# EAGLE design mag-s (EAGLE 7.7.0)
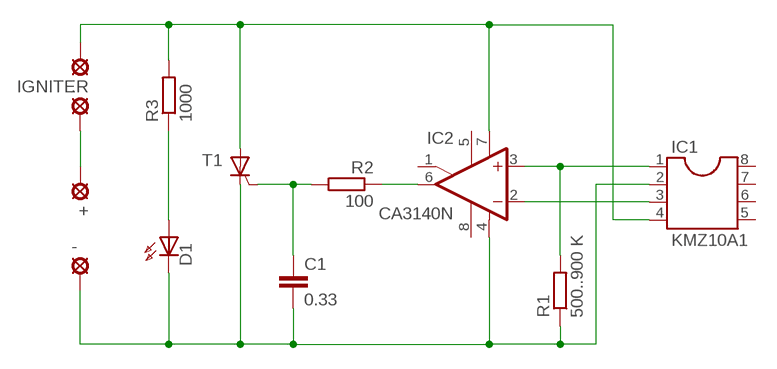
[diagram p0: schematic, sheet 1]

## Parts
+  SE11  [SE11]
-  SE11  [SE11]
.  SE11  [SE11]
C1  0.33  C-EUC0805K  [C0805K]
D1  HLMP6  [HLMP6]
IC1  KMZ10A1  DIL8  [DIL08]
IC2  CA3140N  [DIL08]
IGNITER  SE11  [SE11]
R1  500..900 K  R-EU_M0805  [M0805]
R2  100  R-EU_M0805  [M0805]
R3  1000  R-EU_M0805  [M0805]
T1  BT151  [TO220CL]

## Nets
N$2: IC1.4 IC2.7(V+) IGNITER.MP R3.2 T1.A
N$4: C1.1 R2.2 T1.G
N$5: D1.A R3.1
N$6: -.MP C1.2 D1.K IC1.2 IC2.4(V-) R1.1 T1.C
N$7: IC1.1 IC2.3(+IN) R1.2
N$8: +.MP ..MP
N$9: IC2.6(OUT) R2.1
N$10: IC1.3 IC2.2(-IN)
Unconnected: IC1.5 IC1.6 IC1.7 IC1.8 IC2.1(ON/CMP) IC2.5(ON) IC2.8(CMP)

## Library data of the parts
+ - . IGNITER = solpad:SE11: SOLDER PAD
C1 = rcl:C-EU: CAPACITOR, European symbol
D1 = display-hp:HLMP6: LED
IC1 = ic-package:DIL8: Dual In Line / Socket
IC2 = linear:CA3140: OP AMP
R1-R3 = rcl:R-EU_: RESISTOR, European symbol
T1 = triac:BT151: THYRISTOR

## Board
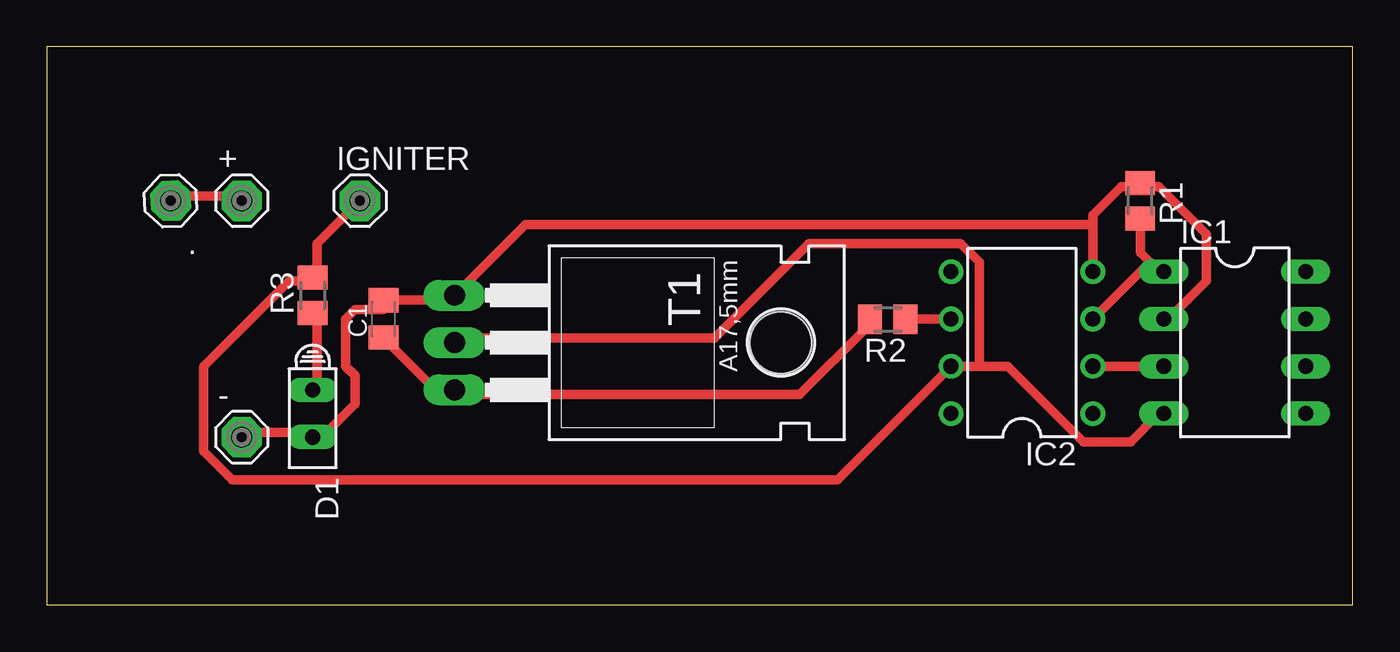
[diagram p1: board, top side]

Size 70.17 x 30.01 mm. Coordinates in mm from the lower left corner, seen from the top.
Outline: 0,0 70.17,0 70.17,30.01 0,30.01 0,0
Copper layers 1: Top 0.035mm
Design rules "default": minimum track width 20mil, minimum drill 20mil, track to track 20mil, track to pad 20mil, pad to pad 20mil, via to via 20mil, smd to smd 25mil, copper to edge 20mil, drill to drill 8mil, minimum pad ring 10mil, minimum via ring 8mil, stop-mask expansion 4mil, vias tented up to drill 0mil, thermal gap 10mil

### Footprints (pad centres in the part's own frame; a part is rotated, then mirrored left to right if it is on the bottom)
SE11 = drill 1.118 pad 2.159 octagon: MP 0,0
C0805K = smd 1.3 x 1.6: 1 -1,0; 2 1,0
HLMP6 = drill 0.813 long: A -1.27,0; K 1.27,0
DIL08 = drill 0.813 long: 1 -3.81,-3.81; 2 -1.27,-3.81; 3 1.27,-3.81; 4 3.81,-3.81; 5 3.81,3.81; 6 1.27,3.81; 7 -1.27,3.81; 8 -3.81,3.81
DIL08' = drill 0.813 pad 1.27: 1 -3.81,-3.81; 2 -1.27,-3.81; 3 1.27,-3.81; 4 3.81,-3.81; 5 3.81,3.81; 6 1.27,3.81; 7 -1.27,3.81; 8 -3.81,3.81
M0805 = smd 1.3 x 1.6: 1 -0.95,0; 2 0.95,0
TO220CL = drill 1.118 long: A 0,-6.35; C -2.54,-6.35; G 2.54,-6.35 | hole 3.302: 0,11.176

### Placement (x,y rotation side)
+  10.48,21.72 0 top
-  10.48,9.02 0 top
.  6.67,21.72 182.6 top
C1  18.1,15.37 90 top
D1  14.29,10.29 270 top
IC1  63.82,14.1 270 top
IC2  CA3140N  [DIL08']  52.39,14.1 90 top
IGNITER  16.83,21.72 0 top
R1  58.74,21.72 270 top
R2  45.18,15.35 180 top
R3  14.29,16.64 90 top
T1  28.26,14.1 270 top

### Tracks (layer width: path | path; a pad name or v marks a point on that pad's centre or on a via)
N$2
  Top 0.508: IGNITER.MP 14.54,19.43 14.54,17.91 R3.2 14.04,17.4 13.02,17.4 8.45,12.83 8.45,8.26 9.97,6.73 42.48,6.73 IC2.7 50.1,12.83 | 50.1,12.83 51.63,12.83 55.69,8.77 58.23,8.77 59.76,10.29 IC1.4 | 50.1,12.83 50.1,18.42 49.09,19.43 40.96,19.43 35.88,14.35 22.16,14.35 T1.A
N$4
  Top 0.508: C1.1 18.1,14.35 20.64,11.81 21.66,11.81 T1.G 22.16,11.31 40.45,11.31 44.01,14.86 R2.2
N$5
  Top 0.508: R3.1 14.54,15.37 14.54,11.81 D1.A
N$6
  Top 0.508: 58.74,22.48 57.72,22.48 56.2,20.96 56.2,20.45 | IC2.4 56.2,20.45 | 58.74,22.48 59.76,22.48 62.3,19.94 62.3,17.4 60.26,15.37 IC1.2 | 58.74,22.48 R1.1 | -.MP 10.48,9.27 14.04,9.27 D1.K 14.54,8.77 16.58,10.8 16.58,12.32 16.07,12.83 16.07,15.37 16.58,15.88 18.1,15.88 C1.2 18.1,16.39 21.66,16.39 T1.C 25.72,20.45 56.2,20.45
N$7
  Top 0.508: R1.2 58.74,18.93 59.25,18.42 | 59.25,18.42 59.76,17.91 IC1.1 59.25,18.42 | 59.25,18.42 IC2.3
N$8
  Top 0.508: ..MP 6.92,21.97 10.48,21.97 +.MP
N$9
  Top 0.508: IC2.6 46.55,15.37 R2.1
N$10
  Top 0.508: IC1.3 IC2.2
